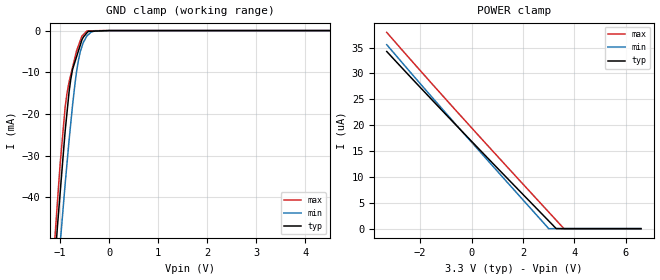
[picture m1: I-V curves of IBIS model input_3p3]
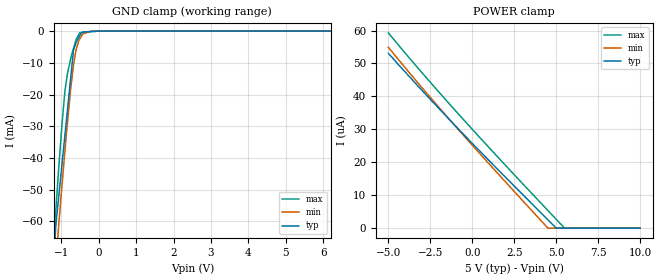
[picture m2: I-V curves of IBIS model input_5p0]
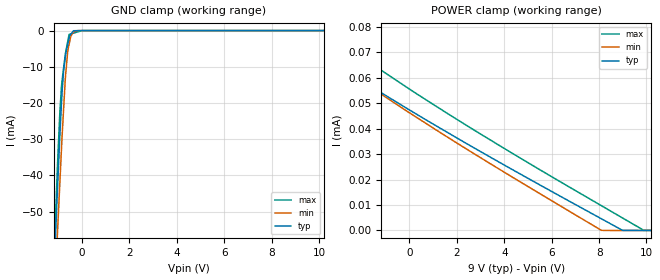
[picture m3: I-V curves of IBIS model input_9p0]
|Texas Instruments Incorporated
| 2.2A Low Voltage Stepper w/ 32-step Indexer or Dual Brushed DC Motor Driver
| (Indexer or PH/EN Ctrl)
| Marketing part#   Digital Voltage Range   Package-type   #pins
| DRV8834PWP   2.5 V - 10.8 V   PWP   24
| DRV8834PWPR   2.5 V - 10.8 V   PWP   24
| DRV8834RGER   2.5 V - 10.8 V   RGE   24
| DRV8834RGET   2.5 V - 10.8 V   RGE   24
[IBIS Ver]   3.2
[File name]   drv8834.ibs
[File Rev]   1.0
[Date]   6/5/2012
[Source]
| Texas Instruments Incorporated.
| Analog-eLab Design Center, HPA
| 12500 TI Blvd
| Dallas, TX -75243
| e-mail: elab_scm_ibis@list.ti.com
[Notes]   Revision History:
| Rev 1.0: 6/5/2012
| - Initial version of the model
| - Model generated from simulations in TISPICE
| - Model matched to SPICE simulation
| - C_comp although listed in numerical order of value are
|   obtained from varying PVT conditions. For PVT conditions for
|   each specific value refer the buffer description under
|   respective [Model]. IBIS model user is responsible for using
|   appropriate C_comp to simulate for Signal Integrity.
| - Model names with a trailing _3p3 contains the model for
|   3.3V [3.0V and 3.6V]. Model names with a trailing _5p0 contains
|   the model for 5.0V [4.5V and 5.5V]. Model names with a
|   trailing _9p0 contains
|   the model for 9.0V [8.1V and 9.9V].
|*   EXCEPTION:   *
|*   - For the model FAULT,leakage current is present  in power clamp IV Table *
|*   due to the pull-down transistors in ESD and buffer cell connected to   *
|*   the pad   *
|*   - For the model INPUT,leakage current is present in power clamp I-V Table *
|*   due to a pulldown resistor connected to the pad   *
|*   - For the model M0_APHASE,leakage current is present in power clamp I-V   *
|*   Table due to a pulldown resistor connected to the pad   *
|*   - For the model SLEEP, leakage current is present in the power clamp I-V  *
|*   Table due to a pulldown resistor and  a diode connected to the pad   *
[Disclaimer]
| This model is designed as an aid for customers of Texas Instruments.
| TI and its licensors and suppliers make no warranties, either expressed
| or implied, with respect to this  model, including the warranties of
| merchantability or fitness for a particular purpose. The model is
| provided solely on an "as is" basis. The entire risk as to its quality
| and performance is with the customer.
[Copyright]
 (C) Copyright 2011 Texas Instruments Incorporated.All rights reserved.
|   DRV8834PWP
[Component]   DRV8834PWP
[Manufacturer]   TI
[Package]   |24 HTSSOP   -  PWP package
|   typ   min   max
R_pkg   0.03891   0.01369   0.05820
L_pkg   1.85997nH   1.35307nH   2.41718nH
C_pkg   0.33834pF   0.25571pF   0.42629pF
[Pin]  signal_name   model_name   R_pin   L_pin   C_pin
1   nSLEEP   SLEEP   0.05102   2.16313nH  0.37705pF
2   BDECAY   TERM   0.05188   2.11027nH  0.34262pF
3   ADECAY   TERM   0.05509   2.19187nH  0.29676pF
4   AOUT1   TERM   0.02072   1.72576nH  0.38837pF
5   AISEN   TERM   0.01396   1.39260nH  0.35310pF
6   AOUT2   TERM   0.01773   1.46884nH  0.33694pF
7   BOUT2   TERM   0.01759   1.44972nH  0.35652pF
8   BISEN   TERM   0.01369   1.35307nH  0.35367pF
9   BOUT1   TERM   0.02182   1.77180nH  0.42629pF
10   nENBL/AENBL   INPUT   0.05820   2.41718nH  0.40573pF
11   STEP/BENBL   INPUT   0.05444   2.28420nH  0.39933pF
12   DIR/BPHASE   INPUT   0.04765   1.96107nH  0.32681pF
13   M0/APHASE   M0_APHASE   0.04746   1.91436nH  0.26419pF
14   M1   INPUT   0.04785   1.92472nH  0.29084pF
15   CONFIG   INPUT   0.05032   2.01113nH  0.28012pF
16   nFAULT   FAULT   0.04332   1.76609nH  0.25571pF
17   VCP   TERM   0.04180   1.71229nH  0.26840pF
18   VM   POWER   0.01929   1.56523nH  0.35363pF
19   VM   POWER   0.02086   1.65499nH  0.41940pF
20   VINT   POWER   0.04949   2.10057nH  0.37656pF
21   GND   GND   0.01748   1.48294nH  0.43255pF
22   AVREF   POWER   0.05440   2.15954nH  0.39790pF
23   BVREF   POWER   0.04975   1.99624nH  0.38703pF
24   VREFO   TERM   0.04586   1.86137nH  0.36775pF
|   DRV8834RGE
[Component]   DRV8834RGE
[Manufacturer]   TI
[Package]   |24 VQFN   -  RGE package
|   typ   min   max
R_pkg   0.02763   0.01008   0.04188
L_pkg   1.17754nH   0.98900nH   1.41385nH
C_pkg   0.19390pF   0.16184pF   0.24924pF
[Pin]  signal_name   model_name   R_pin   L_pin   C_pin
1   AOUT1   TERM   0.01633   1.32994nH  0.24924pF
2   AISEN   TERM   0.01020   1.08660nH  0.24700pF
3   AOUT2   TERM   0.01436   1.26269nH  0.23273pF
4   BOUT2   TERM   0.01430   1.25320nH  0.23131pF
5   BISEN   TERM   0.01008   1.07582nH  0.24365pF
6   BOUT1   TERM   0.01605   1.30983nH  0.24643pF
7   nENBL/AENBL   INPUT   0.04071   1.37295nH  0.17809pF
8   STEP/BENBL   INPUT   0.03369   1.12389nH  0.17674pF
9   DIR/BPHASE   INPUT   0.02976   0.98900nH  0.16321pF
10   M0/APHASE   M0_APHASE   0.03036   1.00524nH  0.16220pF
11   M1   INPUT   0.03209   1.06275nH  0.16723pF
12   CONFIG   INPUT   0.03758   1.25454nH  0.16886pF
13   nFAULT   FAULT   0.03822   1.27565nH  0.16647pF
14   VCP   TERM   0.03787   1.25735nH  0.17676pF
15   VM   POWER   0.01593   1.34801nH  0.24828pF
16   VM   POWER   0.01597   1.34297nH  0.25414pF
17   VINT   POWER   0.04015   1.33665nH  0.18667pF
18   GND   GND   0.01400   1.06360nH  0.22107pF
19   AVREF   POWER   0.04186   1.40285nH  0.18000pF
20   BVREF   POWER   0.03411   1.13060nH  0.17582pF
21   VREFO   TERM   0.02991   0.99074nH  0.16184pF
22   nSLEEP   SLEEP   0.02991   0.99385nH  0.16199pF
23   BDECAY   TERM   0.03411   1.13776nH  0.17618pF
24   ADECAY   TERM   0.04188   1.41385nH  0.18032pF
25   thermal_pad   NC   0.00002   0.00339nH  0.56682pF
|   Model Selectors
[Model Selector] INPUT
input_3p3  3.3V digital input
input_5p0  5.0V digital input
input_9p0  9.0V digital input
[Model Selector] SLEEP
sleep_3p3  3.3V digital input
sleep_5p0  5.0V digital input
sleep_9p0  9.0V digital input
[Model Selector] M0_APHASE
m0_aphase_3p3  3.3V digital input
m0_aphase_5p0  5.0V digital input
m0_aphase_9p0  9.0V digital input
[Model Selector] FAULT
fault_3p3  3.3V digital open_drain
fault_5p0  5.0V digital open_drain
fault_9p0  9.0V digital open_drain
[Model Selector] TERM
term_3-3V  3.3V nominal termination
term_5-0V  5.0V nominal termination
term_9-0V  9.0V nominal termination
[Model] term_3-3V
Model_type Terminator
C_comp   1.0e-20F  1.0e-20F  1.0e-20F
|   typ   min   max
[Voltage Range]   3.3V   3.0V   3.6V
[POWER Clamp Reference]   3.3V   3.0V   3.6V
[GND Clamp Reference]   0V   0V   0V
|Ambient Temperature   25   150   -40
|Junction Temperature
[Temperature Range]   27   125   -40
[Model] term_5-0V
Model_type Terminator
C_comp   1.0e-20F  1.0e-20F  1.0e-20F
|   typ   min   max
[Voltage Range]   5.0V   4.5V   5.5V
[POWER Clamp Reference]   5.0V   4.5V   5.5V
[GND Clamp Reference]   0V   0V   0V
|Ambient Temperature   25   150   -40
|Junction Temperature
[Temperature Range]   27   125   -40
[Model] term_9-0V
Model_type Terminator
C_comp   1.0e-20F  1.0e-20F  1.0e-20F
|   typ   min   max
[Voltage Range]   9.0V   8.1V   9.9V
[POWER Clamp Reference]   9.0V   8.1V   9.9V
[GND Clamp Reference]   0V   0V   0V
|Ambient Temperature   25   150   -40
|Junction Temperature
[Temperature Range]   27   125   -40
| Models and submodels in the file (15): input_3p3 (Input), input_5p0 (Input), input_9p0 (Input), sleep_3p3 (Input), sleep_5p0 (Input), sleep_9p0 (Input), m0_aphase_3p3 (Input), m0_aphase_5p0 (Input), m0_aphase_9p0 (Input), fault_3p3 (Open_drain), fault_5p0 (Open_drain), fault_9p0 (Open_drain), term_3-3V (Terminator), term_5-0V (Terminator), term_9-0V (Terminator)
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|   input_3p3 Model
[Model]   input_3p3
Model_type   Input
Vinl = 0.7
Vinh = 2
|   typ   min   max
|   (nom PVT)   (fast PVT)   (slow PVT)
|C_comp from frequency sweep method (F=250KHz)
|Average
|C_comp   2.691e-12   2.459e-12   2.918e-12
|C_comp from LC tank measurement(L=1nH)
|Average
|Resonant Frequency(Hz)   4.340e+09   4.370e+09   4.270e+09
 C_comp   1.346e-12   1.328e-12   1.391e-12
| Where nom  PVT is Nominal Process, 3.3V, 27C
|   Fast PVT is Strong Process,  3.6V, -40C
|   Slow PVT is Weak Process,   3V, 125C
[Voltage Range]   3.3   3   3.6
|Ambient Temperature   25   150   -40
|Junction Temperature
[Temperature Range]   27   125   -40
[Power Clamp Reference]   3.3   3   3.6
[GND Clamp Reference]   0   0   0
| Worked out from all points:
|   GND clamp passes 1 mA (typ) near -0.49 V on its own axis
[GND Clamp]
|   Voltage   I(typ)   I(min)   I(max)
-3.3V     -460.7mA   -437.6mA   -483mA
-1.166V   -65.08mA   -75.53mA   -59.76mA
-1.065V   -48.72mA   -60.47mA   -42.91mA
-1.001V   -39.19mA   -51.42mA   -32.24mA
-896.4mV  -24.04mA   -36.7mA    -18.29mA
-782.1mV  -11.67mA   -22.16mA   -10.59mA
-690mV    -7.216mA   -12.11mA   -6.106mA
-633mV    -5.109mA   -7.542mA   -3.839mA
-531mV    -1.658mA   -2.973mA   -1.022mA
-453.6mV  -537.9uA   -1.306mA   -112.8uA
-3mV      -15.4nA    -23.96nA   -16.18nA
6.6V      0A         0A         0A
[POWER Clamp]
|   Voltage   I(typ)   I(min)   I(max)
-3.3V     34.23uA    35.55uA    37.92uA
-453.6mV  19.24uA    19.26uA    21.99uA
2.997V    1.544uA    18.86nA    3.25uA
3.297V    16.77nA    0A         1.635uA
3.604V    0A         0A         0A
6.6V      0A         0A         0A
|   input_5p0 Model
[Model]   input_5p0
Model_type   Input
Vinl = 0.7
Vinh = 2
|   typ   min   max
|   (nom PVT)   (fast PVT)   (slow PVT)
|C_comp from frequency sweep method (F=250KHz)
|Average
|C_comp   2.598e-12   2.378e-12   2.824e-12
|C_comp from LC tank measurement(L=1nH)
|Average
|Resonant Frequency(Hz)   4.390e+09   4.440e+09   4.310e+09
 C_comp   1.316e-12   1.286e-12   1.365e-12
| Where nom  PVT is Nominal Process, 5V, 27C
|   Fast PVT is Strong Process,  5.5V, -40C
|   Slow PVT is Weak Process,   4.5V, 125C
[Voltage Range]   5   4.5   5.5
|Ambient Temperature   25   150   -40
|Junction Temperature
[Temperature Range]   27   125   -40
[Power Clamp Reference]   5   4.5   5.5
[GND Clamp Reference]   0   0   0
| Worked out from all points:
|   GND clamp passes 1 mA (typ) near -0.49 V on its own axis
[GND Clamp]
|   Voltage   I(typ)   I(min)   I(max)
-5V       -796.6mA   -746.9mA   -837.8mA
-1.216V   -73.11mA   -83.06mA   -68.4mA
-1.179V   -67.02mA   -77.43mA   -62.1mA
-1.14V    -60.52mA   -71.68mA   -55.37mA
-1.078V   -53.26mA   -62.55mA   -44.66mA
-907.5mV  -33.29mA   -38.37mA   -19.47mA
-836mV    -24.92mA   -28.92mA   -13.44mA
-675mV    -6.062mA   -10.76mA   -5.501mA
-603mV    -3.589mA   -5.768mA   -2.645mA
-506mV    -1.428mA   -2.476mA   -478.5uA
-202.5mV  -141uA     -11.61uA   -191.5uA
10V       0A         0A         0A
[POWER Clamp]
|   Voltage   I(typ)   I(min)   I(max)
-5V       53.09uA    54.87uA    59.28uA
-3.26V    43.28uA    44.22uA    48.74uA
-907.5mV  30.53uA    30.38uA    35.12uA
1.512V    17.86uA    16.65uA    21.63uA
4.495V    2.571uA    29.22nA    5.415uA
4.995V    25.44nA    0A         2.722uA
5.505V    0A         0A         0A
10V       0A         0A         0A
|   input_9p0 Model
[Model]   input_9p0
Model_type   Input
Vinl = 0.7
Vinh = 2
|   typ   min   max
|   (nom PVT)   (fast PVT)   (slow PVT)
|C_comp from frequency sweep method (F=250KHz)
|Average
|C_comp   2.465e-12   2.248e-12   2.685e-12
|C_comp from LC tank measurement(L=1nH)
|Average
|Resonant Frequency(Hz)   4.480e+09   4.550e+09   4.400e+09
 C_comp   1.263e-12   1.225e-12   1.310e-12
| Where nom  PVT is Nominal Process, 9V, 27C
|   Fast PVT is Strong Process,  9.9V, -40C
|   Slow PVT is Weak Process,   8.1V, 125C
[Voltage Range]   9   8.1   9.9
|Ambient Temperature   25   150   -40
|Junction Temperature
[Temperature Range]   27   125   -40
[Power Clamp Reference]   9   8.1   9.9
[GND Clamp Reference]   0   0   0
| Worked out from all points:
|   GND clamp passes 1 mA (typ) near -0.47 V on its own axis
[GND Clamp]
|   Voltage   I(typ)   I(min)   I(max)
-9V       -1.598A    -1.486A    -1.684A
-1.197V   -69.79mA   -80.18mA   -65.59mA
-1.053V   -46.78mA   -58.72mA   -40.68mA
-1.03V    -43.31mA   -55.38mA   -36.76mA
-930.6mV  -28.66mA   -41.73mA   -22.23mA
-861.3mV  -19.76mA   -32.17mA   -15.18mA
-765mV    -10.45mA   -20.54mA   -9.842mA
-696.6mV  -7.116mA   -12.73mA   -6.306mA
-599.4mV  -3.79mA    -5.583mA   -2.97mA
-544.5mV  -2.14mA    -3.839mA   -1.087mA
-360mV    -46.39uA   -328.9uA   -718.4uA
18V       0A         0A         0A
[POWER Clamp]
|   Voltage   I(typ)   I(min)   I(max)
-9V       4.253mA    4.281mA    5.847mA
-2.831V   250.3uA    409.7uA    81.06uA
-2.772V   213uA      374.9uA    73.73uA
-2.583V   108.6uA    264.2uA    72.13uA
-2.439V   63.91uA    181.9uA    70.98uA
-2.219V   60.22uA    80.07uA    69.55uA
-2.138V   59.74uA    63.56uA    69.02uA
-2.025V   59.06uA    59.06uA    68.29uA
8.092V    4.633uA    53.89nA    9.784uA
8.991V    45.85nA    0A         4.91uA
9.89V     0A         0A         53.34nA
18V       0A         0A         0A
